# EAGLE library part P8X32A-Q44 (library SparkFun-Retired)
Propellor uC RETIRED
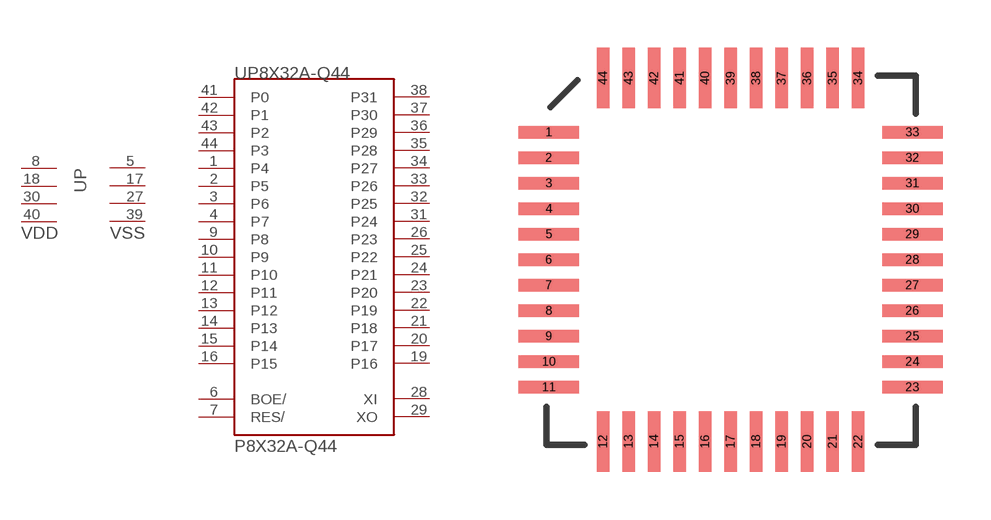
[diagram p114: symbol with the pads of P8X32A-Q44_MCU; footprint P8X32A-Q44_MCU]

Designator prefix U; gates P=4VDD4VSS P8X32A-Q44=P8X32A

## P8X32A-Q44 (PROD_ID: IC-10929; VALUE: P8X32A)  [P8X32A-Q44_MCU]
1  P8X32A-Q44:P4
2  P8X32A-Q44:P5
3  P8X32A-Q44:P6
4  P8X32A-Q44:P7
5  P:VSS  pwr
6  P8X32A-Q44:BOE/  in
7  P8X32A-Q44:RES/
8  P:VDD  pwr
9  P8X32A-Q44:P8
10  P8X32A-Q44:P9
11  P8X32A-Q44:P10
12  P8X32A-Q44:P11
13  P8X32A-Q44:P12
14  P8X32A-Q44:P13
15  P8X32A-Q44:P14
16  P8X32A-Q44:P15
17  P:VSS  pwr
18  P:VDD  pwr
19  P8X32A-Q44:P16
20  P8X32A-Q44:P17
21  P8X32A-Q44:P18
22  P8X32A-Q44:P19
23  P8X32A-Q44:P20
24  P8X32A-Q44:P21
25  P8X32A-Q44:P22
26  P8X32A-Q44:P23
27  P:VSS  pwr
28  P8X32A-Q44:XI  in
29  P8X32A-Q44:XO  out
30  P:VDD  pwr
31  P8X32A-Q44:P24
32  P8X32A-Q44:P25
33  P8X32A-Q44:P26
34  P8X32A-Q44:P27
35  P8X32A-Q44:P28
36  P8X32A-Q44:P29
37  P8X32A-Q44:P30
38  P8X32A-Q44:P31
39  P:VSS  pwr
40  P:VDD  pwr
41  P8X32A-Q44:P0
42  P8X32A-Q44:P1
43  P8X32A-Q44:P2
44  P8X32A-Q44:P3

## Footprint P8X32A-Q44_MCU (pad centres in mm)
smd 1.9 x 0.4: 1 -5.713,4.013; 2 -5.713,3.212; 3 -5.713,2.413; 4 -5.713,1.613; 5 -5.713,0.812; 6 -5.713,0.013; 7 -5.713,-0.787; 8 -5.713,-1.587; 9 -5.713,-2.388; 10 -5.713,-3.188; 11 -5.713,-3.987; 23 5.688,-3.987; 24 5.688,-3.188; 25 5.688,-2.388; 26 5.688,-1.587; 27 5.688,-0.787; 28 5.688,0.013; 29 5.688,0.812; 30 5.688,1.613; 31 5.688,2.413; 32 5.688,3.212; 33 5.688,4.013
smd 0.4 x 1.9: 12 -4.013,-5.688; 13 -3.212,-5.688; 14 -2.413,-5.688; 15 -1.613,-5.688; 16 -0.812,-5.688; 17 -0.013,-5.688; 18 0.787,-5.688; 19 1.587,-5.688; 20 2.388,-5.688; 21 3.188,-5.688; 22 3.987,-5.688; 34 3.987,5.713; 35 3.188,5.713; 36 2.388,5.713; 37 1.587,5.713; 38 0.787,5.713; 39 -0.013,5.713; 40 -0.812,5.713; 41 -1.613,5.713; 42 -2.413,5.713; 43 -3.212,5.713; 44 -4.013,5.713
